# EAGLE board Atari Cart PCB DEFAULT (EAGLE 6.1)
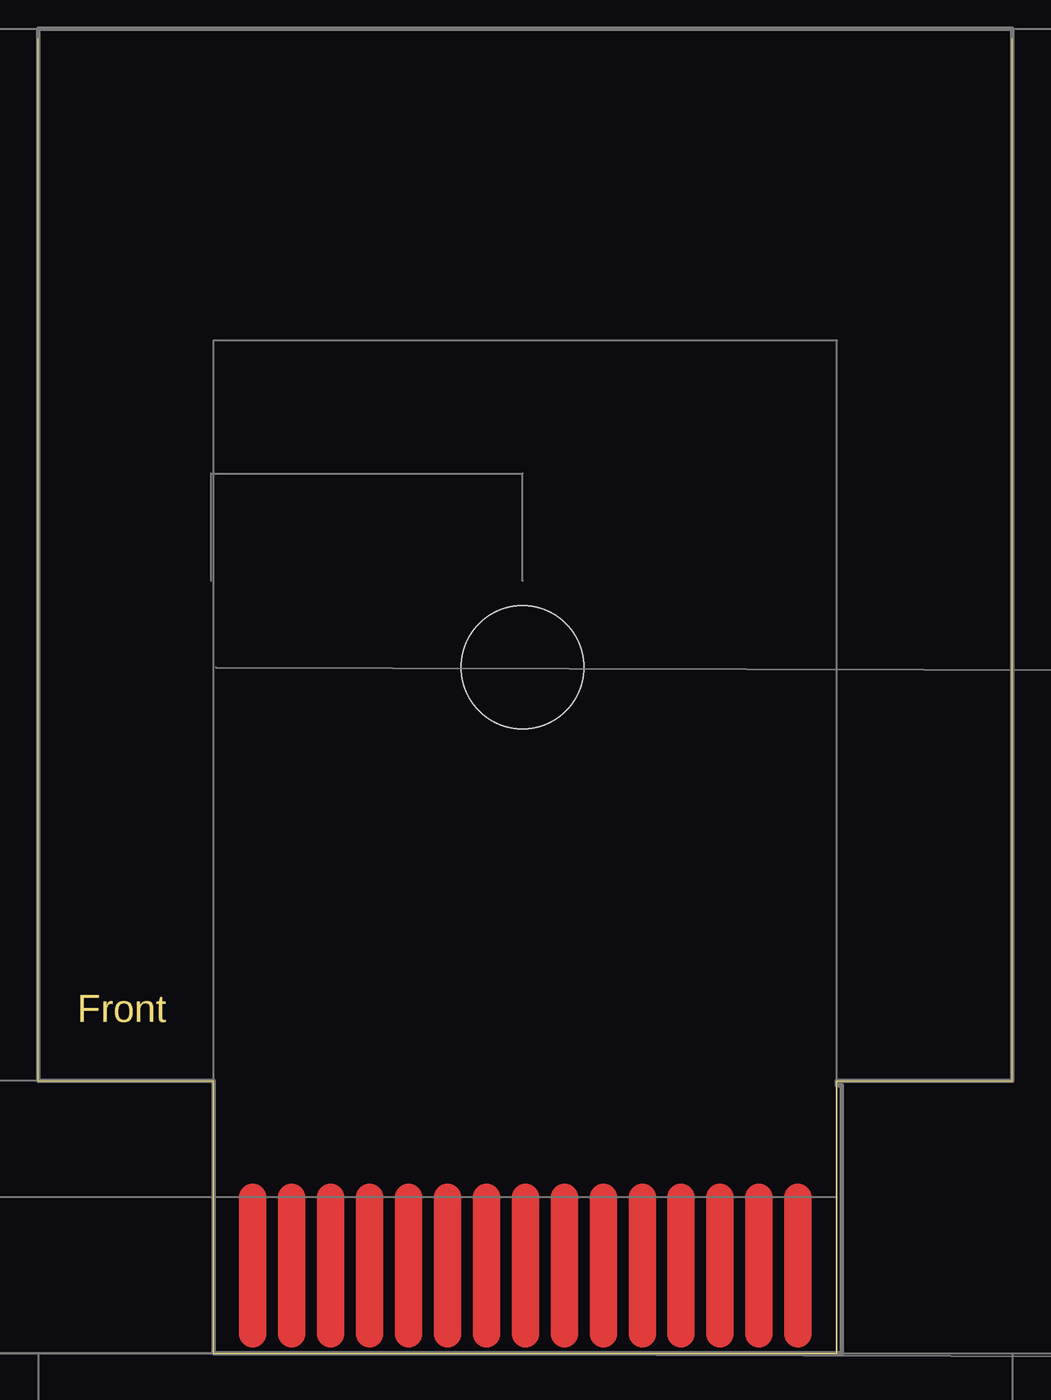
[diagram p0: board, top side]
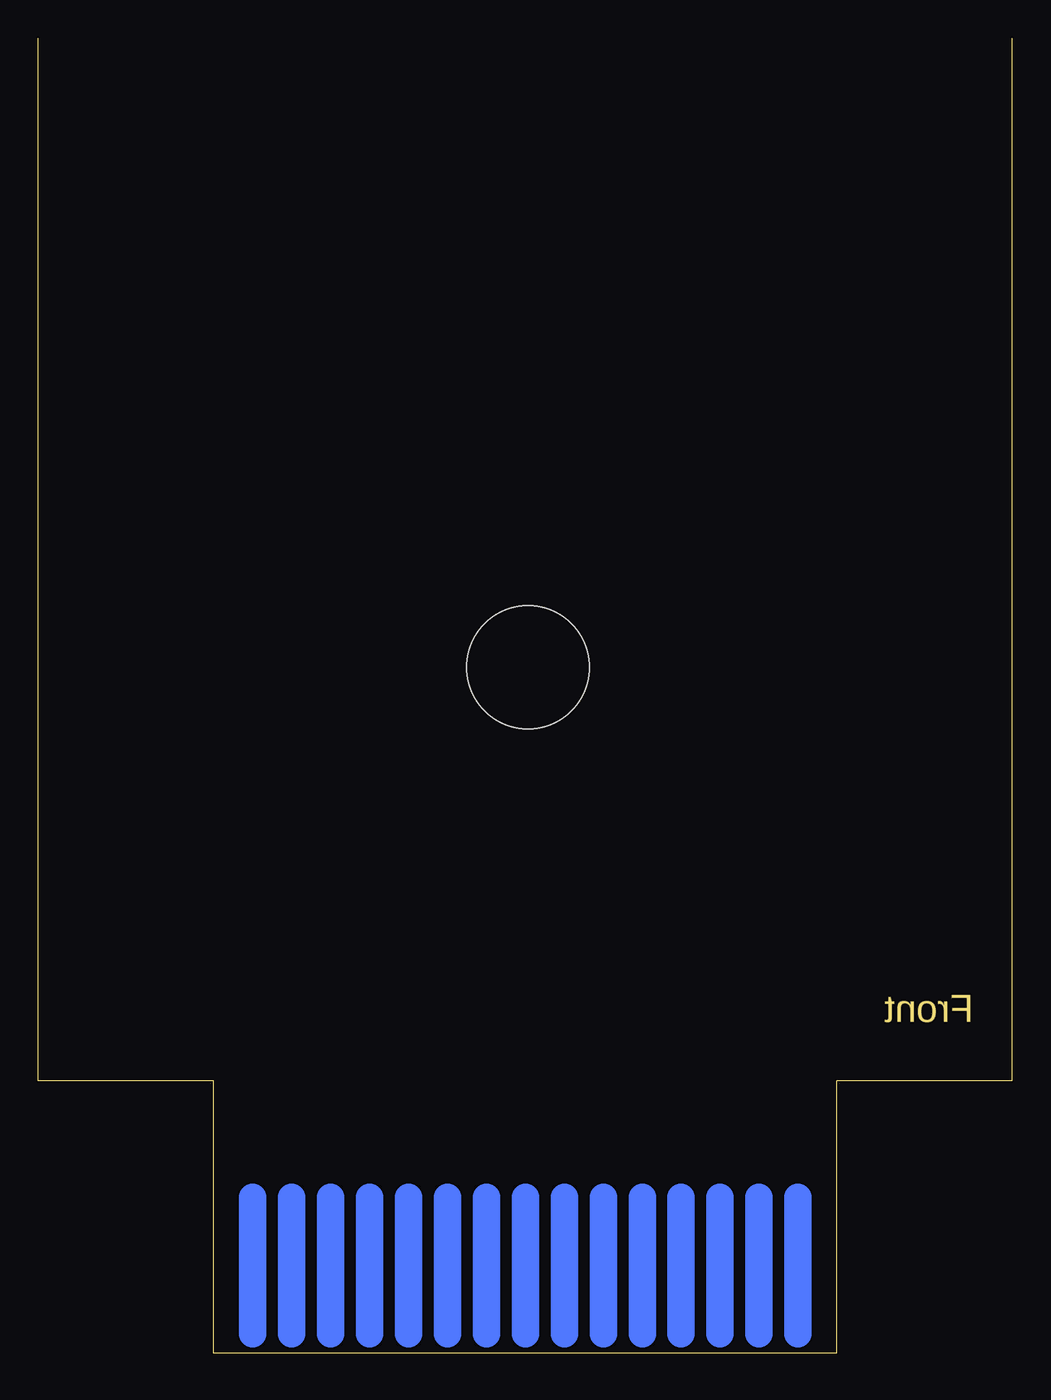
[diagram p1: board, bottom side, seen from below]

Size 63.5 x 85.72 mm. Coordinates in mm from the lower left corner, seen from the top.
Outline: 63.5,85.72 63.5,17.78 52.07,17.78 52.07,0 11.43,0 11.43,17.78 0,17.78 0,85.72
Copper layers (1*16): Top 0.035mm / dielectric 1.5mm / Bottom 0.035mm
Design rules: minimum track width 10mil, minimum drill 24mil, track to track 8mil, track to pad 8mil, pad to pad 8mil, via to via 8mil, smd to smd 8mil, copper to edge 40mil, drill to drill 8mil, minimum pad ring 10mil, minimum via ring 8mil, stop-mask expansion 4mil, vias tented up to drill 0mil, thermal gap 10mil
Holes 8 mm at 31.57,44.72

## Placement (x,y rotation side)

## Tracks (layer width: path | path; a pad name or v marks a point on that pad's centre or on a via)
S$17
  Top 1.778: 16.51,10.16 16.51,1.27
S$31
  Bottom 1.778: 13.97,10.16 13.97,1.27
S$32
  Top 1.778: 13.97,10.16 13.97,1.27
S$33
  Bottom 1.778: 16.51,10.16 16.51,1.27
S$35
  Bottom 1.778: 19.05,10.16 19.05,1.27
S$36
  Top 1.778: 19.05,10.16 19.05,1.27
S$37
  Bottom 1.778: 21.59,10.16 21.59,1.27
S$38
  Top 1.778: 21.59,10.16 21.59,1.27
S$39
  Bottom 1.778: 24.13,10.16 24.13,1.27
S$40
  Top 1.778: 24.13,10.16 24.13,1.27
S$41
  Bottom 1.778: 26.67,10.16 26.67,1.27
S$42
  Top 1.778: 26.67,10.16 26.67,1.27
S$43
  Bottom 1.778: 29.21,10.16 29.21,1.27
S$44
  Top 1.778: 29.21,10.16 29.21,1.27
S$45
  Bottom 1.778: 31.75,10.16 31.75,1.27
S$46
  Top 1.778: 31.75,10.16 31.75,1.27
S$47
  Bottom 1.778: 34.29,10.16 34.29,1.27
S$48
  Top 1.778: 34.29,10.16 34.29,1.27
S$49
  Bottom 1.778: 36.83,10.16 36.83,1.27
S$50
  Top 1.778: 36.83,10.16 36.83,1.27
S$51
  Bottom 1.778: 39.37,10.16 39.37,1.27
S$52
  Top 1.778: 39.37,10.16 39.37,1.27
S$53
  Bottom 1.778: 41.91,10.16 41.91,1.27
S$54
  Top 1.778: 41.91,10.16 41.91,1.27
S$55
  Bottom 1.778: 44.45,10.16 44.45,1.27
S$56
  Top 1.778: 44.45,10.16 44.45,1.27
S$57
  Bottom 1.778: 46.99,10.16 46.99,1.27
S$58
  Top 1.778: 46.99,10.16 46.99,1.27
S$59
  Bottom 1.778: 49.53,10.16 49.53,1.27
S$60
  Top 1.778: 49.53,10.16 49.53,1.27

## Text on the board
Dimension: Front
tDocu: ATARI CARTRIDGE DEFAULT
